(* Logix 5000 Routine export J1939Router; software revision 19.01 *)

TYPE AparianJ1939RInputData :
STRUCT
   InstanceNameLen : DINT;
   InstanceName : SINT[16];
   Status : AparianJ1939RInputStatus;
   TransactionRate : DINT;
   Temperature : REAL;
   RxCANCount : DINT;
   TxCANCount : DINT;
   CANCrcCount : DINT;
   CANBitError : DINT;
   CANStuffError : DINT;
   J1939ReqTxCount : DINT;
   J1939ReqRxCount : DINT;
   J1939ResTxCount : DINT;
   J1939ResRxCount : DINT;
   TagReadCount : DINT;
   TagWriteCount : DINT;
   TagConnFailCount : DINT;
   TagErrorCount : DINT;
   MappedItems : SINT[40];
END_STRUCT
END_TYPE

TYPE AparianJ1939RInputStatus :
STRUCT
   ConfigValid : BOOL;
   DuplicateNode : BOOL;
END_STRUCT
END_TYPE

VAR_GLOBAL   (* controller tags *)
   J1939R01Input : AparianJ1939RInputData;
END_VAR

PROGRAM MainProgram

ROUTINE J1939Router   (* ladder *)
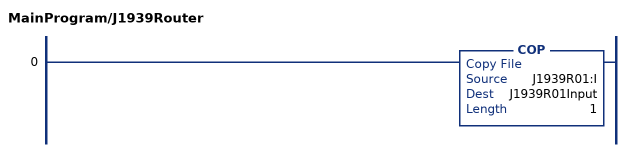
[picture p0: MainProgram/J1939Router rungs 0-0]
   0: COP(J1939R01:I,J1939R01Input,1);
END_ROUTINE
END_PROGRAM
